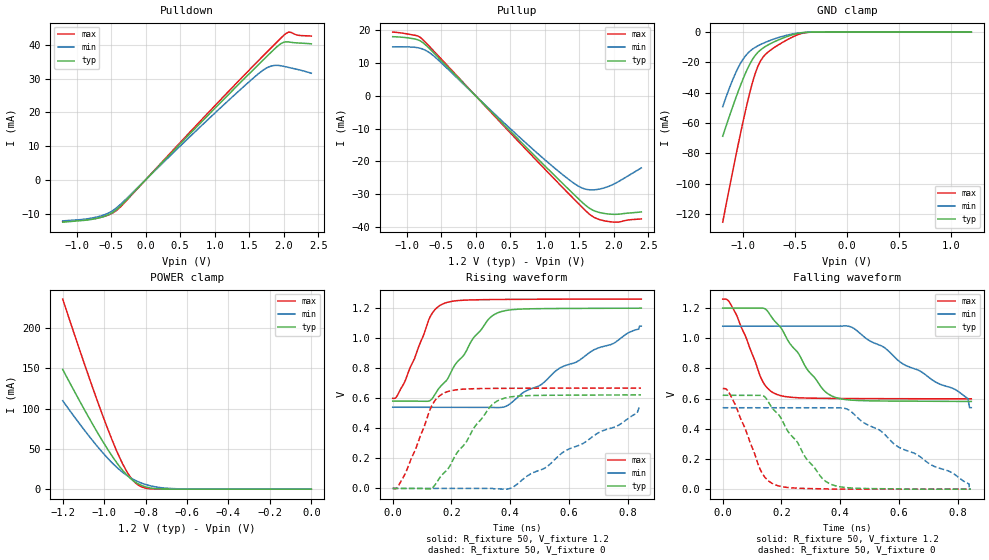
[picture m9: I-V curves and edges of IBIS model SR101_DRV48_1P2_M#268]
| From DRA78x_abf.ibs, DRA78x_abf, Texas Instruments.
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| Model based on original model for DDR_DIFFIOPB_V
|   Sub model SR101_DRV48_1P2
[model]   SR101_DRV48_1P2_M#268
|[Description]  [1.2V-I/O-X-X]
|   , ,
|[Input Load]
|[Output Drive]
|Voltage   1.2V
|Mode   I/O
Model_type   I/O
Polarity   Non-Inverting
Enable   Active-Low
Vinl =  0.47
Vinh =  0.73
Cref =  15.0000pF
Rref =  100.0000M
Vref =  0V
Vmeas =  0.6
C_comp   2p   2p   2p
[Model Spec]
Vinl   0.47   0.41   0.50
Vinh   0.73   0.67   0.76
[Receiver Thresholds]
Tslew_ac = 5n
Vth = 0.6
Vth_max = 0.63
Vth_min = 0.54
Vinh_ac = 0.22
Vinh_dc = 0.13
Vinl_ac = -0.22
Vinl_dc = -0.13
[Temperature Range]   25   125   -40
[Voltage Range]   1.2   1.08   1.26
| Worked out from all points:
|   slope of the pulldown table from 0 to 0.18 V, typ, clamps not added: 46.8 ohm
|   slope of the pullup table from 0 to 0.18 V, typ, clamps not added: 46.2 ohm
|   GND clamp passes 1 mA (typ) near -0.48 V on its own axis
|   POWER clamp passes 1 mA (typ) near -0.76 V on its own axis
|   rising waveform, R_fixture 50, V_fixture 1.2: 20-80 % time 131ps typ, 305ps min, 78.7ps max; typ from 0.581 V to 1.2 V
|   rising waveform, R_fixture 50, V_fixture 0: 20-80 % time 129ps typ, 296ps min, 79ps max; typ from 0 V to 0.622 V
|   falling waveform, R_fixture 50, V_fixture 1.2: 20-80 % time 130ps typ, 290ps min, 79.2ps max; typ from 1.2 V to 0.581 V
|   falling waveform, R_fixture 50, V_fixture 0: 20-80 % time 131ps typ, 294ps min, 78.6ps max; typ from 0.622 V to 0 V
[POWER_clamp]
-1.2V     148.6mA    109.7mA    235.9mA
-1.115V   108mA      79.97mA    170.5mA
-1.055V   80.16mA    59.93mA    125.3mA
-1.006V   59.04mA    45.03mA    90.73mA
-957.6mV  39.59mA    31.69mA    58.49mA
-921.2mV  26.75mA    23.11mA    36.96mA
-897mV    19.41mA    18.26mA    24.7mA
-860.6mV  10.74mA    12.35mA    10.83mA
-836.4mV  6.696mA    9.316mA    5.268mA
-787.9mV  2.052mA    4.939mA    818.3uA
-666.7mV  49.08uA    692.2uA    5.202uA
0V        48.89nA    205.6nA    269.9nA
[Pulldown]
-1.2V     -12.53mA   -12.14mA   -12.38mA
-690.9mV  -11.33mA   -10.92mA   -11.28mA
-509.1mV  -10.05mA   -9.509mA   -10.14mA
-400mV    -8.43mA    -7.908mA   -8.698mA
1.018V    21.49mA    20.06mA    22.27mA
1.527V    31.95mA    29.55mA    33.07mA
1.745V    36.35mA    33.05mA    37.6mA
1.855V    38.51mA    33.85mA    39.84mA
1.964V    40.39mA    33.77mA    42.05mA
2.073V    40.83mA    33.28mA    43.75mA
2.218V    40.52mA    32.6mA     42.79mA
2.4V      40.27mA    31.57mA    42.58mA
[Pullup]
-1.2V     18.06mA    14.95mA    19.46mA
-836.4mV  17.11mA    14.68mA    18.27mA
-763.6mV  16.25mA    14.25mA    17.17mA
-654.5mV  14.13mA    12.98mA    14.77mA
836.4mV   -17.91mA   -16.46mA   -18.74mA
1.273V    -27.02mA   -24.3mA    -28.28mA
1.527V    -32.21mA   -28.03mA   -33.73mA
1.636V    -34.17mA   -28.69mA   -35.95mA
1.709V    -35.05mA   -28.74mA   -37.06mA
1.855V    -35.92mA   -28.18mA   -38.15mA
2.036V    -36.22mA   -26.61mA   -38.62mA
2.4V      -35.49mA   -22.03mA   -37.62mA
[GND_clamp]
-1.2V     -68.74mA   -49.24mA   -125.5mA
-1.127V   -53.92mA   -35.5mA    -100.1mA
-1.055V   -39.92mA   -23.99mA   -75.5mA
-981.8mV  -27.37mA   -15.83mA   -52.4mA
-909.1mV  -17.63mA   -11.09mA   -32.41mA
-860.6mV  -13.38mA   -9.079mA   -22.59mA
-836.4mV  -11.86mA   -8.241mA   -19.18mA
-787.9mV  -9.515mA   -6.746mA   -14.76mA
-739.4mV  -7.652mA   -5.419mA   -11.95mA
-521.2mV  -1.657mA   -1.168mA   -3.09mA
-375.8mV  -108.2uA   -128.9uA   -198.1uA
1.2V      48.89nA    308.5nA    224.4nA
[Ramp]
dV/dt_f 0.37190929/0.1299015n 0.32528022/0.29143166n 0.39705855/79.326079p
dV/dt_r 0.37562096/0.13054649n 0.32695279/0.30025466n  0.4025516/79.323354p
R_load = 50
[Rising Waveform]
R_fixture = 50
V_fixture = 1.2
V_fixture_min = 1.08
V_fixture_max = 1.26
0s        581.3mV    540.1mV    599.2mV
13.2ps    581.2mV    540.1mV    609.9mV
40ps      580.7mV    540.1mV    704.9mV
123.9ps   581.6mV    540mV      1.127V
171ps     694.5mV    540.1mV    1.228V
275.7ps   1.003V     539.9mV    1.255V
357ps     1.168V     537.8mV    1.257V
501.1ps   1.196V     685mV      1.259V
569ps     1.197V     800.8mV    1.259V
846.6ps   1.2V       1.08V      1.26V
[Rising Waveform]
R_fixture = 50
V_fixture = 0
V_fixture_min = 0
V_fixture_max = 0
0s        0V         0V         0V
15.3ps    0V         0V         6.567mV
41.9ps    0V         0V         94.77mV
133.7ps   0V         0V         552.7mV
178.1ps   109.2mV    0V         638.1mV
279.8ps   412.3mV    0V         663.8mV
363.2ps   589mV      -3.717mV   665.9mV
409.3ps   611.3mV    8.414mV    666.3mV
779.4ps   621.6mV    433.1mV    667.6mV
845.3ps   622.4mV    539.9mV    667.6mV
[Falling Waveform]
R_fixture = 50
V_fixture = 1.2
V_fixture_min = 1.08
V_fixture_max = 1.26
0s        1.2V       1.08V      1.26V
43.7ps    1.2V       1.08V      1.168V
137.2ps   1.2V       1.08V      710.3mV
180.7ps   1.106V     1.08V      630.6mV
335.3ps   676.3mV    1.08V      602.1mV
382.6ps   608.8mV    1.081V     601.3mV
447.1ps   589.1mV    1.065V     600.5mV
616.9ps   583.6mV    826.6mV    599.5mV
800.1ps   582.3mV    650.7mV    599.1mV
846.6ps   581.3mV    540.1mV    599mV
[Falling Waveform]
R_fixture = 50
V_fixture = 0
V_fixture_min = 0
V_fixture_max = 0
0s        622.4mV    539.9mV    667.2mV
42.5ps    622.6mV    540mV      561.8mV
131.6ps   621.7mV    540mV      114.9mV
175.3ps   523.3mV    540mV      31.3mV
285.7ps   199.7mV    540mV      4.063mV
371.4ps   30.2mV     540.2mV    0V
428.2ps   9.084mV    526.1mV    0V
595.5ps   2.074mV    283mV      0V
782.5ps   0V         107.2mV    0V
845.3ps   0V         0V         0V
